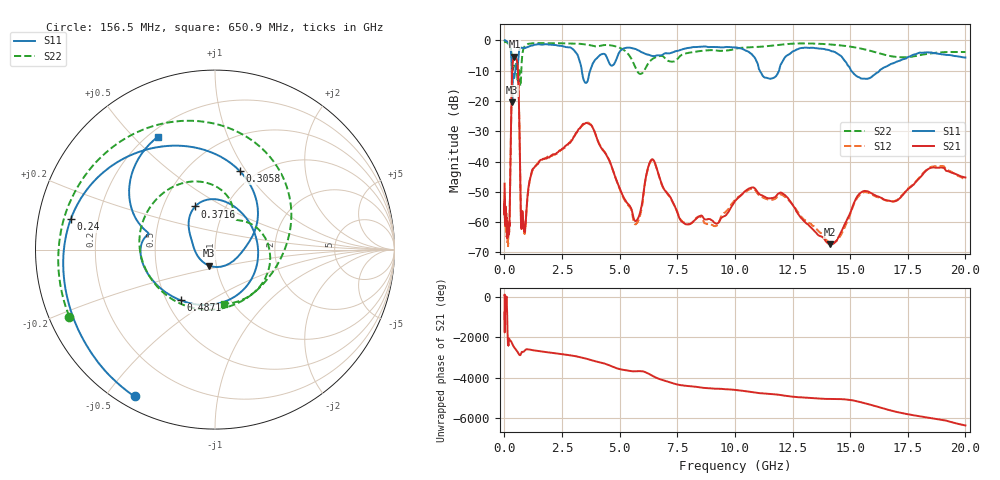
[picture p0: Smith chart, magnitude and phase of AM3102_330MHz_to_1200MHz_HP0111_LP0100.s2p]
! Date/Time: Tue, Sep 11, 2018 5:15 PM
! Network Analyzer: Agilent Technologies E8362B Rev: A.07.50.63
! Sweep from 0.010 to 20.000 GHz, 1601 Points, Sweep Type: LOG
! Power Supply: 4.949 V, 0.001 A
# Hz S DB R 50
!freq MagS11 AngS11 MagS21 AngS21 MagS12 AngS12 MagS22 AngS22
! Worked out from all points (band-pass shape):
!   1601 points, 10 MHz to 20 GHz, reference 50 ohm
!   highest |S21| = -5.42 dB at 438.8 MHz (marker M1); lowest = -67.3 dB at 14.14 GHz (marker M2)
!   |S21| within 3 dB of the highest: 349.6 MHz to 577.6 MHz (228 MHz wide, 49.2 % of centre)
!   lowest |S11| = -20.4 dB at 341.1 MHz (marker M3), VSWR 1.21, Z = 46.2 - j8.33 ohm
!   |S11| at or under -10 dB: 3.36 GHz to 3.719 GHz (359.4 MHz wide, 10.2 % of centre); 11.08 GHz to 11.92 GHz (834.8 MHz wide, 7.26 % of centre); 15.04 GHz to 16.28 GHz (1.231 GHz wide, 7.86 % of centre)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
!   |S22| runs from -15.1 to -0.2 dB; largest |S21 - S12| = 0.0082
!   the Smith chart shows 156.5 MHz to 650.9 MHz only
!   S11 on the Smith chart (normalised r, x): 156.5 MHz: 0.05, -0.59; 240 MHz: 0.10, +0.10; 305.8 MHz: 0.84, +0.94; 371.6 MHz: 0.72, +0.37; 487.1 MHz: 0.59, -0.38; 650.9 MHz: 0.24, +0.59
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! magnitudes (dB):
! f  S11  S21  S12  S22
! 10 MHz  0.0  -47.3  -53.7  -0.2
! 35.55 MHz  0.0  -58.9  -59.7  -0.4
! 126.4 MHz  -0.4  -64.0  -63.3  -0.8
! 156.5 MHz  -0.6  -62.6  -67.7  -1.0
! 240 MHz  -1.7  -52.4  -52.4  -1.8
! 305.8 MHz  -6.7  -20.4  -20.4  -4.3
! 341.1 MHz  -20.4  -9.6  -9.7  -8.5
! 371.6 MHz  -11.5  -6.8  -6.8  -9.8
! 438.8 MHz  -11.9  -5.4  -5.5  -7.7
! 447.2 MHz  -11.5  -5.4  -5.5  -7.5
! 487.1 MHz  -9.3  -5.6  -5.7  -7.3
! 650.9 MHz  -3.0  -27.9  -27.9  -10.3
! 726 MHz  -2.4  -61.2  -59.5  -11.7
! 873.8 MHz  -2.5  -63.4  -63.7  -2.0
! 1.59 GHz  -1.4  -39.4  -39.5  -0.9
! 3.668 GHz  -11.4  -27.6  -27.3  -1.5
! 5.652 GHz  -2.7  -59.5  -60.6  -8.4
! 6.426 GHz  -5.2  -39.2  -39.6  -6.1
! 7.845 GHz  -2.7  -60.6  -60.4  -4.3
! 10.79 GHz  -5.0  -48.5  -48.9  -2.3
! 14.14 GHz  -3.4  -67.3  -66.8  -1.3
! 20 GHz  -5.6  -45.3  -45.9  -3.8
